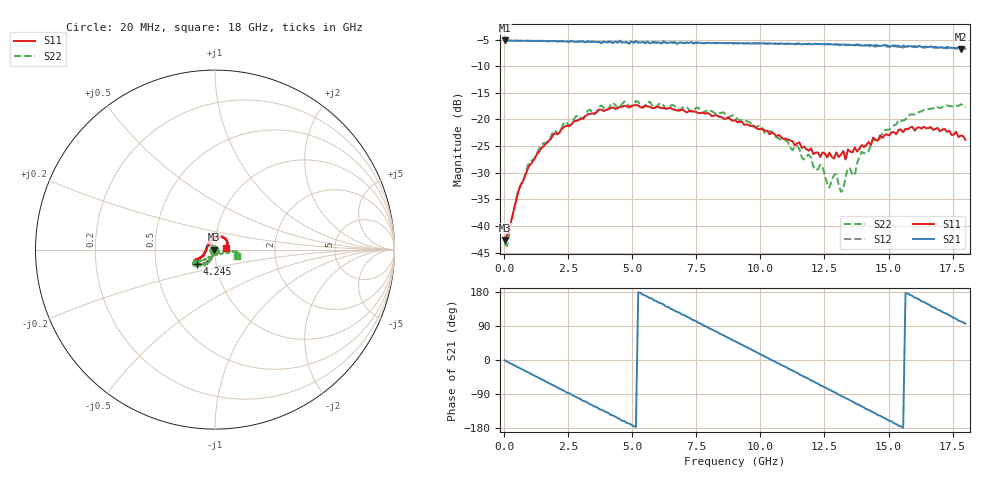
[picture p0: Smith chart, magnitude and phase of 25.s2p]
!Agilent Technologies,N5230A,US43500223,A.07.50.48
!Agilent N5230A: A.07.50.48
!Date: Wednesday, February 17, 2016 11:01:06
!Correction: S11(Full 2 Port(1,2))
!S21(Full 2 Port(1,2))
!S12(Full 2 Port(1,2))
!S22(Full 2 Port(1,2))
!S2P File: Measurements: S11, S21, S12, S22:
# Hz S  RI  R 50
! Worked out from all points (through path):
!   201 points, 20 MHz to 18 GHz, reference 50 ohm
!   highest |S21| = -5.18 dB at 20 MHz (marker M1); lowest = -6.8 dB at 17.82 GHz (marker M2)
!   group delay of S21, straight-line fit = 96.1 ps
!   lowest |S11| = -42.6 dB at 20 MHz (marker M3), VSWR 1.01, Z = 49.3 - j0.0102 ohm
!   |S11| at or under -10 dB: start of sweep to end of sweep
!   |S22| runs from -43.8 to -16.5 dB; largest |S21 - S12| = 0.032
!   S11 on the Smith chart (normalised r, x): 20 MHz: 0.99, -0.00; 4.245 GHz: 0.81, -0.13; 18 GHz: 1.14, +0.02
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2e7  -0.0074 -0.000103  0.5509 -0.00694  0.5493 -0.00762  -0.00687 -6.07e-05
1.0089e9  -0.0131 -0.0353  0.4446 -0.3163  0.4441 -0.3164  -0.0116 -0.0387
2.3574e9  -0.0463 -0.0722  0.0735 -0.5355  0.0729 -0.5333  -0.0494 -0.0809
3.0766e9  -0.0653 -0.0778  -0.1664 -0.514  -0.1624 -0.5152  -0.0633 -0.0796
4.2453e9  -0.1011 -0.0811  -0.4316 -0.2897  -0.4371 -0.2927  -0.1034 -0.0994
5.1443e9  -0.1159 -0.0724  -0.5382 -0.0315  -0.5448 -0.0292  -0.1212 -0.0872
6.0433e9  -0.1147 -0.0622  -0.4629 0.2551  -0.4599 0.2673  -0.1205 -0.0709
7.5716e9  -0.1005 -0.0559  -0.0789 0.5224  -0.0723 0.5173  -0.1061 -0.0747
9.01e9  -0.0859 -0.048  0.3371 0.3954  0.3448 0.389  -0.0844 -0.066
1.05383e10  -0.0653 -0.0336  0.5109 -0.0262  0.5129 -0.0386  -0.0468 -0.0535
1.20666e10  -0.0473 -0.00225  0.285 -0.4214  0.2724 -0.4325  -0.0136 -0.0333
1.23363e10  -0.0442 0.00523  0.205 -0.4686  0.1932 -0.4731  -0.0164 -0.0339
1.26959e10  -0.0444 0.0203  0.1013 -0.4973  0.0915 -0.4987  -0.00378 -0.0226
1.29656e10  -0.0412 0.0268  0.019 -0.5061  -0.00459 -0.5088  0.00767 -0.0297
1.31454e10  -0.0331 0.0332  -0.0384 -0.4991  -0.0528 -0.5035  0.0103 -0.0183
1.34151e10  -0.031 0.0423  -0.1201 -0.4895  -0.1353 -0.4808  0.0226 -0.0266
1.36848e10  -0.0244 0.049  -0.2002 -0.4614  -0.2007 -0.4491  0.0246 -0.0175
1.39545e10  -0.0184 0.0547  -0.2653 -0.4166  -0.2769 -0.4143  0.0463 -0.0183
1.50333e10  0.0111 0.07  -0.4494 -0.1601  -0.4653 -0.1463  0.08 -0.00854
1.6202e10  0.0497 0.0684  -0.4609 0.1724  -0.4348 0.1884  0.1169 -0.0123
1.78202e10  0.0694 0.0143  -0.0924 0.4484  -0.0725 0.4558  0.1358 -0.0264
1.8e10  0.064 0.0089  -0.0485 0.4598  -0.026 0.4609  0.1251 -0.0352
